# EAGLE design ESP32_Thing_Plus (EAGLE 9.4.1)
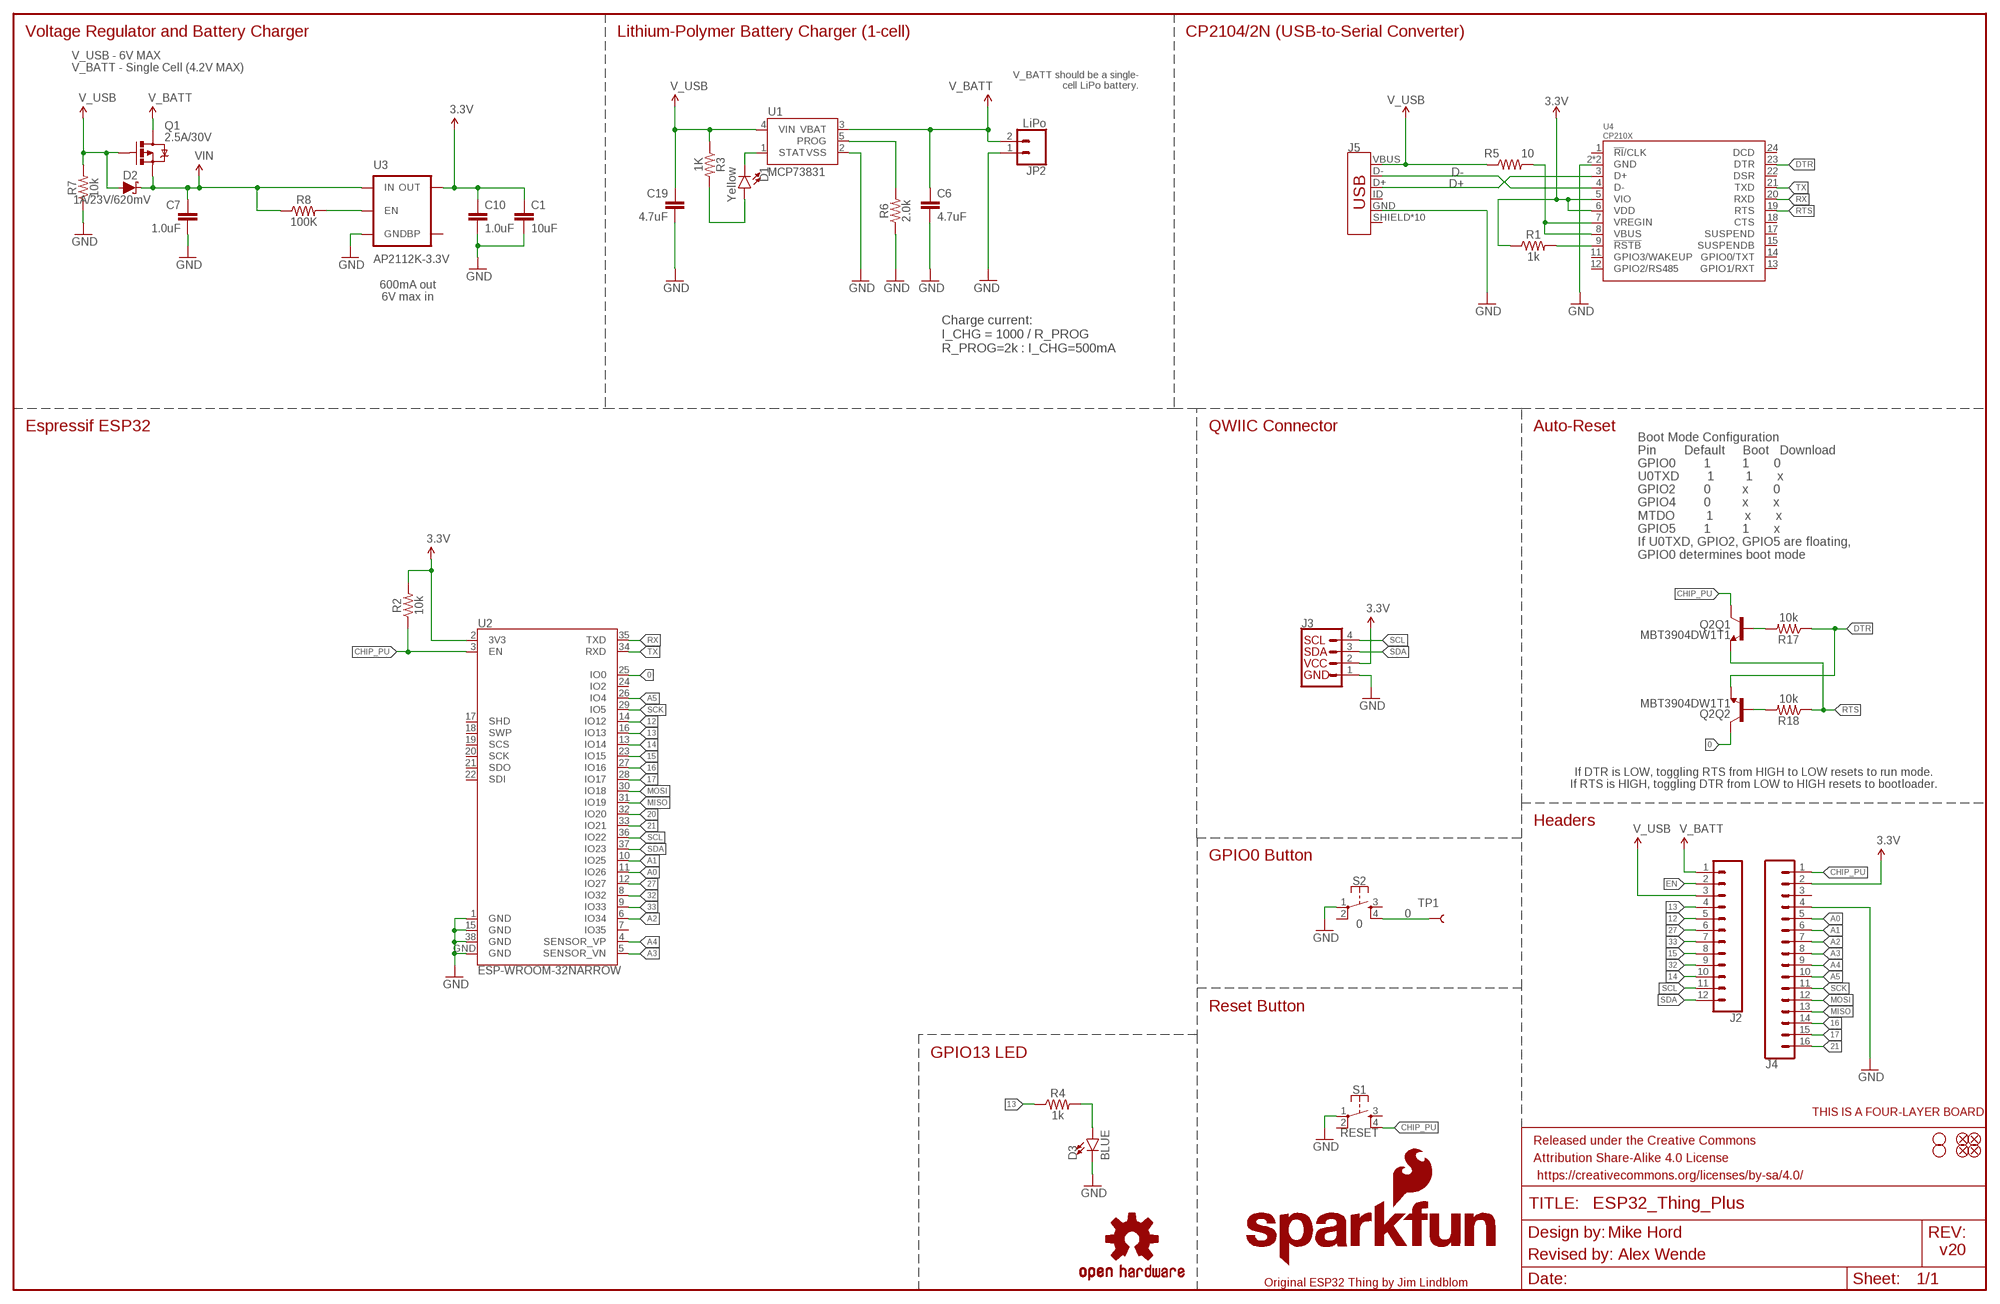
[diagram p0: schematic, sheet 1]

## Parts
C1  10uF  10UF-0603-6.3V-20%  [0603]
C6  4.7uF  4.7UF0603  [0603]
C7  1.0uF  1.0UF-0603-16V-10%-X7R  [0603]
C10  1.0uF  1.0UF-0402-16V-10%  [0402]
C19  4.7uF  4.7UF0603  [0603]
D1  Yellow  LED-YELLOW0603  [LED-0603]
D2  1A/23V/620mV  DIODE-SCHOTTKY-BAT20J  [SOD-323]
D3  BLUE  LED-BLUE0603  [LED-0603]
FD1  FIDUCIALUFIDUCIAL  [FIDUCIAL-MICRO]
FD2  FIDUCIALUFIDUCIAL  [FIDUCIAL-MICRO]
FD3  FIDUCIALUFIDUCIAL  [FIDUCIAL-MICRO]
FD4  FIDUCIALUFIDUCIAL  [FIDUCIAL-MICRO]
FRAME1  FRAME-LEDGER  [CREATIVE_COMMONS]
H1  STAND-OFFTIGHT  [STAND-OFF-TIGHT]
H2  STAND-OFFTIGHT  [STAND-OFF-TIGHT]
J2  CONN_12SM_SQ_NO_SILK  [1X12_SM_SQ_NOSILK]
J3  QWIIC_CONNECTORJS-1MM  [1X04_1MM_RA]
J4  CONN_161X16_SM_SQ_NOSILK  [1X16_SM_SQ_NOSILK]
J5  USB_MICRO-B_HALF_PTH_MILL  [USB-MICROB-PTH-MILL]
JP2  LiPo  CONN_02-JST-2MM-SMT  [JST-2-SMD]
LOGO1  SFE_LOGO_FLAME.1_INCH  [SFE_LOGO_FLAME_.1]
LOGO2  OSHW-LOGOMINI  [OSHW-LOGO-MINI]
LOGO3  SFE_LOGO_NAME_FLAME.1_INCH  [SFE_LOGO_NAME_FLAME_.1]
LOGO4  FOUR_LAYER_WARNING  [FOUR_LAYER_WARNING]
Q1  2.5A/30V  MOSFET-PCHANNELDMG2307L  [SOT23-3@1]
Q2  MBT3904DW1T1  TRANS_NPN_DUAL-MBT3904DW1T1  [SC70-6]
R1  1k  1KOHM-0603-1/10W-1%  [0603]
R2  10k  10KOHM-0603-1/10W-1%  [0603]
R3  1K  1KOHM-1/10W-1%(0603)  [0603]
R4  1k  1KOHM-0603-1/10W-1%  [0603]
R5  10  10OHM-0603-1/10W-5%  [0603]
R6  2.0k  2.0KOHM1/10W5%(0603)  [0603]
R7  10k  10KOHM-0603-1/10W-1%  [0603]
R8  100K  100KOHM-0402-1/16W-1%  [0402]
R17  10k  10KOHM-0603-1/10W-1%  [0603]
R18  10k  10KOHM-0603-1/10W-1%  [0603]
S1  RESET  MOMENTARY-SWITCH-SPST-2-SMD-4.6X2.8MM  [TACTILE_SWITCH_SMD_4.6X2.8MM]
S2  0  MOMENTARY-SWITCH-SPST-2-SMD-4.6X2.8MM  [TACTILE_SWITCH_SMD_4.6X2.8MM]
TP1  TEST-POINTTP_15TH_THRU  [TP_15TH]
U1  MCP73831  [SOT23-5]
U2  ESP-WROOM-32NARROW  [ESP-WROOM-32-NARROW]
U3  AP2112K-3.3V  V_REG_LDOSMD  [SOT23-5]
U4  CP210X  CP2102N  [QFN24]

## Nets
0: Q2.6(Q2:C) S2.4 TP1.P$1 U2.25(IO0)
3.3V: C1.1 C10.1 J3.2 J4.2 R1.1 R2.2 U2.2(3V3) U3.5(OUT) U4.5(VIO) U4.6(VDD)
12: J2.5 U2.14(IO12)
13: J2.4 R4.1 U2.16(IO13)
14: J2.10 U2.13(IO14)
15: J2.8 U2.23(IO15)
16: J4.14 U2.27(IO16)
17: J4.15 U2.28(IO17)
20: U2.32(IO20)
21: J4.16 U2.33(IO21)
27: J2.6 U2.12(IO27)
32: J2.9 U2.8(IO32)
33: J2.7 U2.9(IO33)
A0: J4.5 U2.11(IO26)
A1: J4.6 U2.10(IO25)
A2: J4.7 U2.6(IO34)
A3: J4.8 U2.5(SENSOR_VN)
A4: J4.9 U2.4(SENSOR_VP)
A5: J4.10 U2.26(IO4)
CHG: D1.C U1.1(STAT)
CHIP_PU: J4.1 Q2.3(Q1:C) R2.1 S1.4 U2.3(EN)
D+: J5.D+ U4.3(D+)
D-: J5.D- U4.4(D-)
DTR: Q2.1(Q2:E) R17.1 U4.23(DTR)
EN: J2.2 R8.2 U3.3(EN)
GND: C1.2 C6.2 C7.2 C10.2 C19.2 D3.C J3.1 J4.4 J5.GND JP2.1 R6.1 R7.1 S1.1 S2.1 U1.2(VSS) U2.1(GND) U2.15(GND) U2.38(GND) U2.GND U3.2(GND) U4.2(GND) U4.PAD(GND)
MISO: J4.13 U2.31(IO19)
MOSI: J4.12 U2.30(IO18)
N$1: R1.2 U4.9(!RSTB)
N$2: D3.A R4.2
N$3: R5.2 U4.7(VREGIN) U4.8(VBUS)
N$10: Q2.5(Q1:B) R17.2
N$12: Q2.2(Q2:B) R18.2
N$14: R6.2 U1.5(PROG)
N$17: D1.A R3.2
RTS: Q2.4(Q1:E) R18.1 U4.19(RTS)
RX: U2.35(TXD) U4.20(RXD)
SCK: J4.11 U2.29(IO5)
SCL: J2.11 J3.4 U2.36(IO22)
SDA: J2.12 J3.3 U2.37(IO23)
TX: U2.34(RXD) U4.21(TXD)
V_BATT: C6.1 J2.1 JP2.2 Q1.3(D) U1.3(VBAT)
V_USB: C19.1 D2.A J2.3 J5.VBUS Q1.1(G) R3.1 R5.1 R7.2 U1.4(VIN)
VIN: C7.1 D2.C Q1.2(S) R8.1 U3.1(IN)
Unconnected: J4.3 J5.ID J5.SHIELD J5.SHIELD2(SHIELD) J5.SHIELD3(SHIELD) J5.SHIELD4(SHIELD) J5.SHIELD5(SHIELD) J5.SHIELD6(SHIELD) J5.SHIELD7(SHIELD) J5.SHIELD8(SHIELD) J5.SHIELD9(SHIELD) J5.SHIELD10(SHIELD) S1.2 S1.3 S2.2 S2.3 U2.7(IO35) U2.17(SHD) U2.18(SWP) U2.19(SCS) U2.20(SCK) U2.21(SDO) U2.22(SDI) U2.24(IO2) U3.4(BP) U4.1(!RI!/CLK) U4.11(GPIO3/WAKEUP) U4.12(GPIO2/RS485) U4.13(GPIO1/RXT) U4.14(GPIO0/TXT) U4.15(SUSPENDB) U4.17(SUSPEND) U4.18(CTS) U4.22(DSR) U4.24(DCD)

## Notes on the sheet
- Voltage Regulator and Battery Charger | Lithium-Polymer Battery Charger (1-cell) | CP2104/2N (USB-to-Serial Converter)
- V_USB - 6V MAX
  V_BATT - Single Cell (4.2V MAX)
- V_BATT should be a single-
  cell LiPo battery.
- 600mA out
  6V max in
- Charge current:
  I_CHG = 1000 / R_PROG
  R_PROG=2k : I_CHG=500mA
- Espressif ESP32 | QWIIC Connector | Auto-Reset
- Boot Mode Configuration
  Pin        Default     Boot   Download
  GPIO0        1         1       0
  U0TXD        1         1       x
  GPIO2        0         x       0
  GPIO4        0         x       x
  MTDO         1         x       x
  GPIO5        1         1       x
  If U0TXD, GPIO2, GPIO5 are floating, 
  GPIO0 determines boot mode
- If DTR is LOW, toggling RTS from HIGH to LOW resets to run mode.
  If RTS is HIGH, toggling DTR from LOW to HIGH resets to bootloader.
- Headers
- GPIO0 Button
- Reset Button
- GPIO13 LED
- Mike Hord
- v20
- Revised by: Alex Wende
- Original ESP32 Thing by Jim Lindblom

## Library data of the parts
C1 = SparkFun-Capacitors:10UF: 10.0µF ceramic capacitors; PROD_ID: CAP-11015
C6 C19 = SparkFun-Capacitors:4.7UF: 4.7µF ceramic capacitors; PROD_ID: CAP-08280
C7 = SparkFun-Capacitors:1.0UF: 1µF ceramic capacitors; PROD_ID: CAP-13930
C10 = SparkFun-Capacitors:1.0UF: 1µF ceramic capacitors; PROD_ID: CAP-12417
D1 = SparkFun-LED:LED-YELLOW: Yellow SMD LED; PROD_ID: DIO-09003
D2 = SparkFun-DiscreteSemi:DIODE-SCHOTTKY: Schottky diode; PROD_ID: DIO-11623
D3 = SparkFun-LED:LED-BLUE: Blue SMD LED; PROD_ID: DIO-08575
FD1-FD4 = SparkFun-Aesthetics:FIDUCIAL: Fiducial Alignment Points
FRAME1 = SparkFun-Aesthetics:FRAME-LEDGER: Schematic Frame - Ledger
H1 H2 = SparkFun-Hardware:STAND-OFF: Stand Off
J2 = SparkFun-Connectors:CONN_12: Multi connection point. Often used as Generic Header-pin footprint for 0.1 inch spaced/style header connections On any of the 0.1 inch spaced packages, you can populate with these: Break Away Headers - Straight (PRT-00116) Break Away Male Headers - Right Angle (PRT-00553) Female Headers (PRT-00115)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
J3 = SparkFun-Connectors:QWIIC_CONNECTOR: SparkFun I2C Standard Qwiic Connector An SMD 1mm pitch JST connector makes it easy and quick (get it? Qwiic?) to connect I2C devices to each other. The Qwiic system enables fast and solderless connection between popular platforms and various sensors and actuators. We carry 200mm, 100mm, 50mm, and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; PROD_ID: CONN-13694
J4 = SparkFun-Connectors:CONN_16: Multi connection point. Often used as Generic Header-pin footprint for 0.1 inch spaced/style header connections On any of the 0.1 inch spaced packages, you can populate with these: Break Away Headers - Straight (PRT-00116) Break Away Male Headers - Right Angle (PRT-00553) Female Headers (PRT-00115)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
J5 = SparkFun-Connectors:USB_MICRO-B: USB Type Micro-B Connector Male/female and PTH/SMT variants SparkFun Products: SparkFun microB USB Breakout SparkFun USB microB Plug Breakout SparkFun ESP8266 Thing; PROD_ID: CONN-13711
JP2 = SparkFun-Connectors:CONN_02: Multi connection point. Often used as Generic Header-pin footprint for 0.1 inch spaced/style header connections; PROD_ID: CONN-11443
LOGO1 = SparkFun-Aesthetics:SFE_LOGO_FLAME: SparkFun Flame Logo
LOGO2 = SparkFun-Aesthetics:OSHW-LOGO: Open-Source Hardware (OSHW) Logo
LOGO3 = SparkFun-Aesthetics:SFE_LOGO_NAME_FLAME: SparkFun Font Logo w/ Flame
LOGO4 = SparkFun-Aesthetics:FOUR_LAYER_WARNING: Four-Layer Board Warning - tDoc Layer
Q1 = SparkFun-DiscreteSemi:MOSFET-PCHANNEL: Generic PMOSFET IRLML2244 - TRANS-11153 (SOT-23 -20V -4.3A) (1.Gate 2.Source 3.Drain) FQP27P06 - COM-10349 (TO-220 -60V -27A) (1.Gate 2.Source 3.Drain); PROD_ID: TRANS-11308
Q2 = SparkFun-DiscreteSemi:TRANS_NPN_DUAL: Dual NPN Transistors in Single Package The MBT3904W1 puts two general purpose 3904 NPN transistors in a single package. Datasheet SparkFun Products: SparkFun ESP32 Thing; PROD_ID: TRANS-13337
R1 R4 = SparkFun-Resistors:1KOHM: 1kΩ resistor; PROD_ID: RES-07856
R2 R7 R17 R18 = SparkFun-Resistors:10KOHM: 10kΩ resistor; PROD_ID: RES-00824
R3 = SparkFun-Resistors:1KOHM-1/10W-1%(0603): RES-07856; PROD_ID: RES-07856
R5 = SparkFun-Resistors:10OHM: 10Ω resistor; PROD_ID: RES-09834
R6 = SparkFun-Resistors:2.0KOHM1/10W5%(0603): RES-08296; PROD_ID: RES-08296
R8 = SparkFun-Resistors:100KOHM: 100kΩ resistor; PROD_ID: RES-13495
S1 S2 = SparkFun-Switches:MOMENTARY-SWITCH-SPST-2: Momentary Switch (Pushbutton) - SPST - Two Circuits Normally-open (NO) SPST momentary switches (buttons, pushbuttons). Schematic symbol includes two switch circuits. Variants SMD-4.6MMX2.8MM - 4.60mm x 2.80mm Tactile Momentary Button Switch - Used on SparkFun SAMD21 Mini Breakout SMD-5.2MM - Mini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; PROD_ID: SWCH-13065
TP1 = SparkFun-Connectors:TEST-POINT: SparkFun Test Points
U1 = SparkFun-PowerIC:MCP73831: Miniature single cell, fully integrated Li-Ion, Li-polymer charge management controller http://ww1.microchip.com/downloads/en/DeviceDoc/20001984g.pdf IC-09995; PROD_ID: IC-09995
U2 = SparkFun-RF:ESP-WROOM-32; PROD_ID: IC-13849
U3 = SparkFun-PowerIC:V_REG_LDO: Voltage Regulator LDO Standard 150mA LDO voltage regulator in SOT-23 layout. Micrel part MIC5205. BP (by-pass) pin is used to lower output noise with 470pF cap.; PROD_ID: VREG-12457
U4 = SparkFun-IC-Comms:CP2102N; PROD_ID: IC-14020

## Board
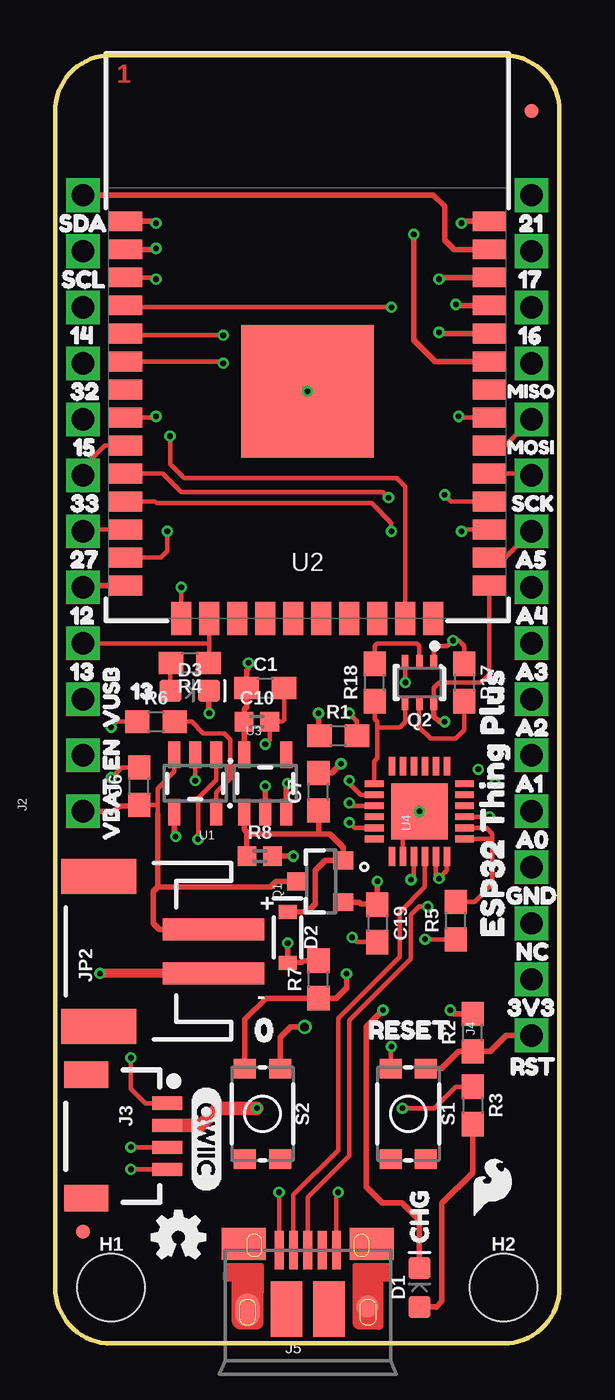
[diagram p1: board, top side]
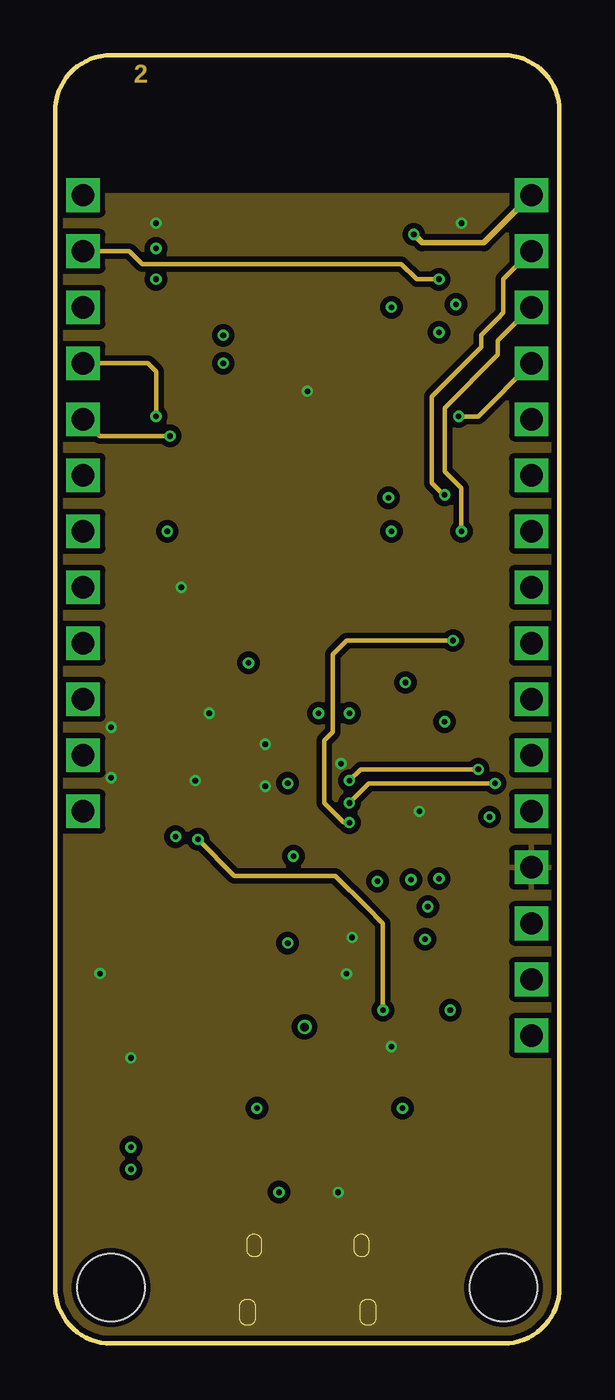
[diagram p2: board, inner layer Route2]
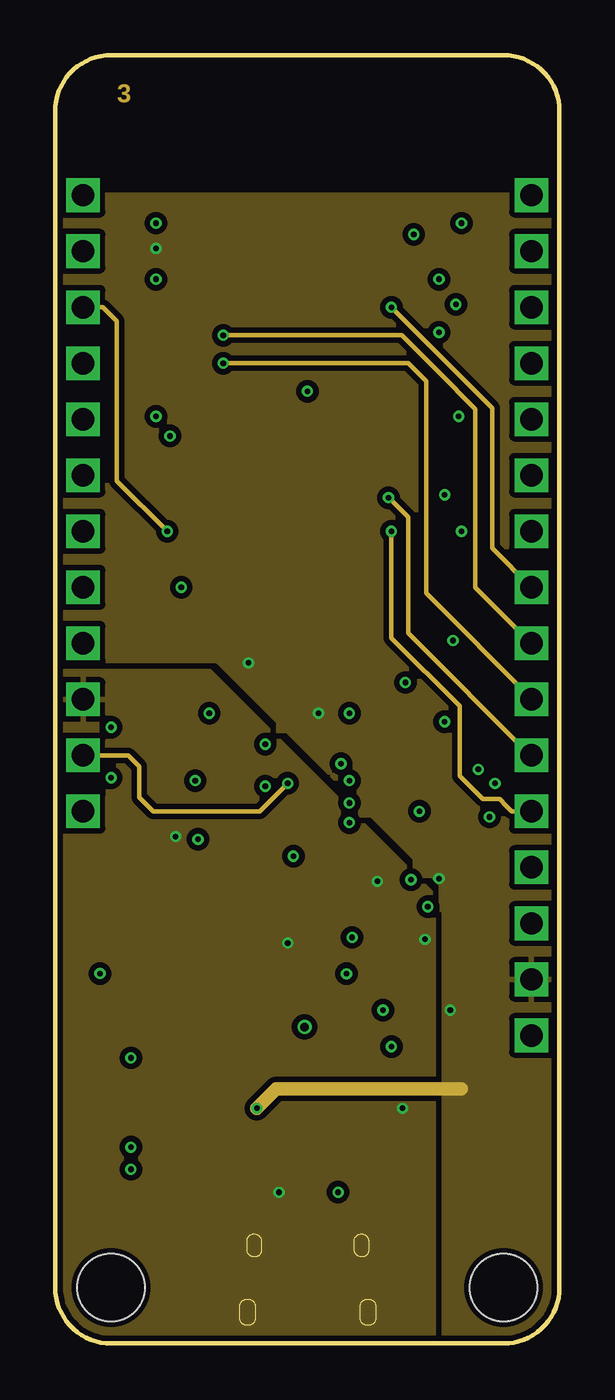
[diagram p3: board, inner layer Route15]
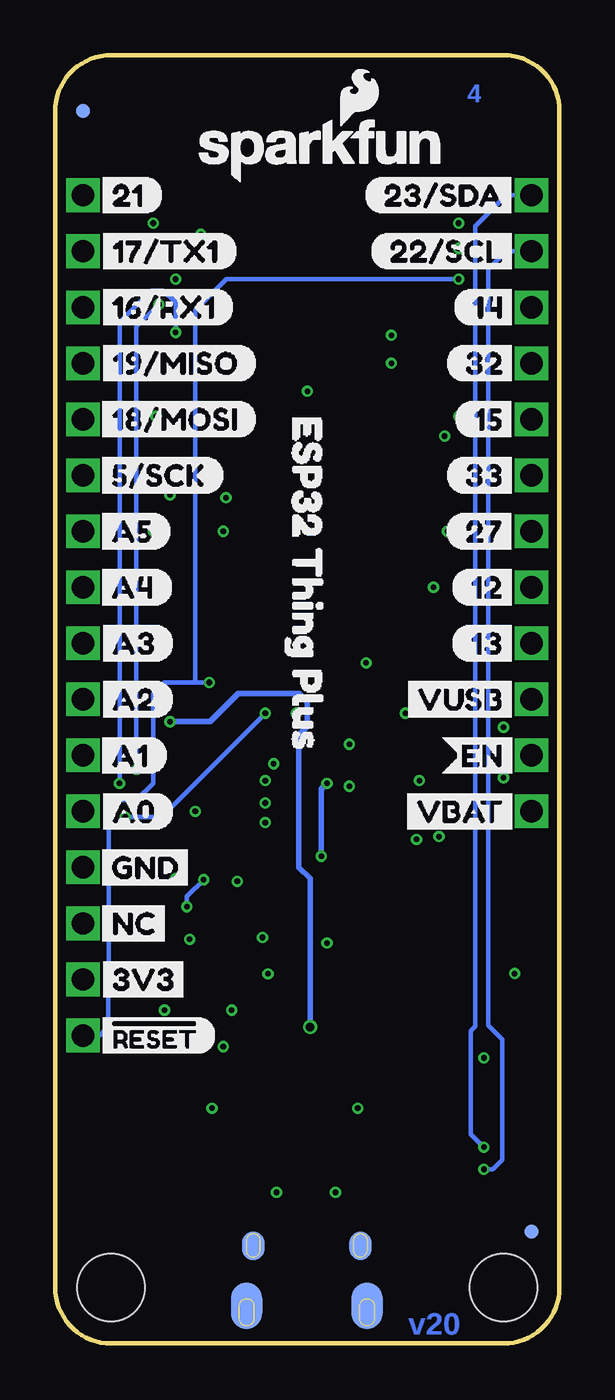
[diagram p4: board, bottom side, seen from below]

Size 22.86 x 58.42 mm. Coordinates in mm from the lower left corner, seen from the top.
Outline: 22.86,2.54 22.86,55.88 arc90 20.32,58.42 2.54,58.42 arc90 0,55.88 0,2.54 arc90 2.54,0 20.32,0 arc90 22.86,2.54
Copper layers (1*2*15*16): Top 0.035559375mm / dielectric 0.47751875mm / Route2 0.035559375mm / dielectric 0.47751875mm / Route15 0.035559375mm / dielectric 0.47751875mm / Bottom 0.035559375mm
Design rules "SparkFun-4-layer-FAB-LIMIT": minimum track width 4mil, minimum drill 6mil, track to track 5mil, track to pad 5mil, pad to pad 5mil, via to via 5mil, smd to smd 5mil, copper to edge 4mil, drill to drill 4mil, minimum pad ring 5mil, minimum via ring 5mil, stop-mask expansion 4mil, vias tented up to drill 25mil, thermal gap 10mil

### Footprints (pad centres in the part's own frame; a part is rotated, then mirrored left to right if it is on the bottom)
0603 = smd 1.1 x 1: 1 -0.85,0; 2 0.85,0
0402 = smd 0.85 x 0.9: 1 -0.58,0; 2 0.58,0
LED-0603 = smd 1 x 1: A -0.877,0; C 0.877,0
SOD-323 = smd 0.63 x 0.83: A 1.15,0; C -1.15,0
FIDUCIAL-MICRO = smd 0.635 x 0.635: 1 0,0
STAND-OFF-TIGHT = hole 3.048: 0,0
1X12_SM_SQ_NOSILK = drill 1.016 pad 1.27 square: 1 0,0; 2 2.54,0; 3 5.08,0; 4 7.62,0; 5 10.16,0; 6 12.7,0; 7 15.24,0; 8 17.78,0; 9 20.32,0; 10 22.86,0; 11 25.4,0; 12 27.94,0
1X04_1MM_RA = smd 0.6 x 1.35: 1 -1.5,0; 2 -0.5,0; 3 0.5,0; 4 1.5,0 | smd 1.2 x 2: NC1 2.8,-3.675; NC2 -2.8,-3.675
1X16_SM_SQ_NOSILK = drill 1.016 pad 1.27 square: 1 0,0; 2 2.54,0; 3 5.08,0; 4 7.62,0; 5 10.16,0; 6 12.7,0; 7 15.24,0; 8 17.78,0; 9 20.32,0; 10 22.86,0; 11 25.4,0; 12 27.94,0; 13 30.48,0; 14 33.02,0; 15 35.56,0; 16 38.1,0
USB-MICROB-PTH-MILL = smd 0.4 x 1.75: D+ 0,0; D- -0.65,0; GND 1.3,0; ID 0.65,0; VBUS -1.3,0 | smd 2 x 1.46: SHIELD -2.9,0.275; SHIELD2 2.9,0.275 | smd 1.425 x 2.5: SHIELD3 -0.963,-2.675; SHIELD4 0.963,-2.675 | smd 1.4 x 2.1 bottom: SHIELD5 -2.731,-2.531; SHIELD7 2.729,-2.531 | smd 1 x 1: SHIELD6 2.7,-2.575 | smd 1.1 x 1.5: SHIELD8 -2.731,-2.731 | smd 1 x 1.3 bottom: SHIELD9 -2.43,0.195; SHIELD10 2.43,0.195
JST-2-SMD = smd 1 x 4.6: 1 -1,-3.7; 2 1,-3.7 | smd 1.6 x 3.4: NC1 -3.4,1.5; NC2 3.4,1.5
SOT23-3@1 = smd 0.8 x 0.9: 1 -0.95,-1; 2 0.95,-1; 3 0,1.1
SC70-6 = smd 0.3 x 0.66: 1 -0.65,-0.92; 2 0,-0.92; 3 0.65,-0.92; 4 0.65,0.92; 5 0,0.92; 6 -0.65,0.92
TACTILE_SWITCH_SMD_4.6X2.8MM = smd 0.9 x 1: 1 -2.05,-0.8; 2 2.05,-0.8; 3 2.05,0.8; 4 -2.05,0.8
TP_15TH = drill 0.381 pad 0.61: P$1 0,0
SOT23-5 = smd 0.55 x 1.2: 1 -0.95,-1.3; 2 0,-1.3; 3 0.95,-1.3; 4 0.95,1.3; 5 -0.95,1.3
ESP-WROOM-32-NARROW = smd 0.9 x 1.5: 1 6.43,8.238; 2 5.16,8.238; 3 3.89,8.238; 4 2.62,8.238; 5 1.35,8.238; 6 0.08,8.238; 7 -1.19,8.238; 8 -2.46,8.238; 9 -3.73,8.238; 10 -5,8.238; 11 -6.27,8.238; 12 -7.54,8.238; 13 -8.81,8.238; 14 -10.08,8.238; 25 -10.08,-8.238; 26 -8.81,-8.238; 27 -7.54,-8.238; 28 -6.27,-8.238; 29 -5,-8.238; 30 -3.73,-8.238; 31 -2.46,-8.238; 32 -1.19,-8.238; 33 0.08,-8.238; 34 1.35,-8.238; 35 2.62,-8.238; 36 3.89,-8.238; 37 5.16,-8.238; 38 6.43,-8.238 | smd 1.5 x 0.9: 15 -11.57,5.715; 16 -11.57,4.445; 17 -11.57,3.175; 18 -11.57,1.905; 19 -11.57,0.635; 20 -11.57,-0.635; 21 -11.57,-1.905; 22 -11.57,-3.175; 23 -11.57,-4.445; 24 -11.57,-5.715 | smd 6 x 6: GND -1.27,0
QFN24 = smd 0.85 x 0.3: 1 -2.05,1.25; 2 -2.05,0.75; 3 -2.05,0.25; 4 -2.05,-0.25; 5 -2.05,-0.75; 6 -2.05,-1.25; 13 2.05,-1.25; 14 2.05,-0.75; 15 2.05,-0.25; 16 2.05,0.25; 17 2.05,0.75; 18 2.05,1.25 | smd 0.3 x 0.85: 7 -1.25,-2.05; 8 -0.75,-2.05; 9 -0.25,-2.05; 10 0.25,-2.05; 11 0.75,-2.05; 12 1.25,-2.05; 19 1.25,2.05; 20 0.75,2.05; 21 0.25,2.05; 22 -0.25,2.05; 23 -0.75,2.05; 24 -1.25,2.05 | smd 2.55 x 2.55: PAD 0,0

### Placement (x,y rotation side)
C1  9.53,29.72 0 top
C6  3.81,25.27 90 top
C7  11.94,25.02 90 top
C10  9.14,28.19 0 top
C19  14.61,19.05 270 top
D1  16.51,2.54 90 top
D2  10.54,18.41 270 top
D3  6.1,29.59 0 top
FD1  21.59,55.88 0 top
FD2  21.59,55.88 0 bottom
FD3  1.27,5.08 0 top
FD4  1.27,5.08 0 bottom
FRAME1  not placed on the board
H1  2.54,2.54 0 top
H2  20.32,2.54 0 top
J2  1.27,24.13 90 top
J3  5.08,9.4 270 top
J4  21.59,13.97 90 top
J5  11.45,4.24 0 top
JP2  3.48,17.78 90 top
LOGO1  18.67,5.46 0 top
LOGO2  5.59,4.83 0 top
LOGO3  16.76,52.58 0 bottom
LOGO4  not placed on the board
Q1  12.06,20.95 90 top
Q2  16.51,29.97 180 top
R1  12.83,27.56 0 top
R2  18.92,14.1 90 top
R3  18.92,10.79 270 top
R4  6.1,30.86 180 top
R5  18.16,19.18 90 top
R6  4.57,28.19 0 top
R7  11.94,16.51 90 top
R8  9.27,22.1 0 top
R17  18.54,29.97 270 top
R18  14.48,29.97 90 top
S1  16,10.41 270 top
S2  9.4,10.41 270 top
TP1  11.3,14.35 0 top
U1  6.35,25.4 180 top
U2  11.43,44.45 90 top
U3  9.53,25.4 0 top
U4  16.51,24.13 90 top
U$1  [#RESET0]  21.34,13.97 0 bottom
U$2  [3V31]  21.21,16.51 0 bottom
U$3  [1323]  4.93,31.75 0 bottom
U$4  [1417]  4.88,46.99 0 bottom
U$5  [1519]  4.83,41.91 0 bottom
U$6  [16#RX11]  21.21,46.99 0 bottom
U$7  [17#TX10]  21.21,49.53 0 bottom
U$8  [121]  4.93,34.29 0 bottom
U$9  [210]  21.18,52.07 0 bottom
U$10  [2721]  5.18,36.83 0 bottom
U$11  [3218]  5.21,44.45 0 bottom
U$12  [3320]  5.21,39.37 0 bottom
U$13  [A03]  21.21,24.13 0 bottom
U$14  [A14]  21.21,26.67 0 bottom
U$15  [A25]  21.21,29.21 0 bottom
U$16  [A36]  21.21,31.75 0 bottom
U$17  [A47]  21.21,34.29 0 bottom
U$18  [A58]  21.21,36.83 0 bottom
U$19  [EN26]  5.38,26.67 0 bottom
U$20  [GND2]  21.21,21.59 0 bottom
U$21  [22#SCL1]  8.64,49.53 0 bottom
U$22  [23#SDA0]  8.86,52.07 0 bottom
U$23  [QWIIC27]  6.86,11.68 270 top
U$27  [VBAT25]  7.39,24.13 0 bottom
U$28  [VUSB24]  7.37,29.21 0 bottom
U$29  [SDA1]  -0.51,50.8 0 top
U$30  [SCL0]  -0.38,48.26 0 top
U$31  [142]  0,45.72 0 top
U$32  [323]  0,43.18 0 top
U$33  [154]  0,40.64 0 top
U$34  [335]  0,38.1 0 top
U$35  [276]  0,35.56 0 top
U$36  [127]  0,33.02 0 top
U$37  [138]  0,30.48 0 top
U$38  [219]  20.19,50.8 0 top
U$39  [1710]  20.32,48.26 0 top
U$40  [1611]  20.32,45.72 0 top
U$41  [A515]  20.19,35.56 0 top
U$42  [A416]  20.07,33.02 0 top
U$43  [A317]  20.07,30.48 0 top
U$44  [A218]  20.07,27.94 0 top
U$45  [A119]  20.19,25.4 0 top
U$46  [A020]  20.19,22.86 0 top
U$47  [SCK20]  20.07,38.1 0 top
U$48  [GND21]  19.76,20.32 0 top
U$49  [NC22]  20.19,17.78 0 top
U$50  [VUSB8]  2.54,27.3 90 top
U$51  [EN9]  2.54,25.4 90 top
U$52  [VBAT10]  2.54,22.23 90 top
U$53  [137]  2.79,29.59 0 top
U$54  [MISO0]  19.94,43.18 0 top
U$55  [MOSI1]  19.94,40.64 0 top
U$56  [CHG1]  16.51,3.81 90 top
U$57  [RESET0]  13.46,14.22 0 top
U$58  [ESP32_THING_PLUS0]  19.81,17.53 90 top
U$59  [ORDERING_INSTRUCTIONS]  not placed on the board
U$60  [3V323]  19.81,15.24 0 top
U$61  [RST24]  19.94,12.57 0 top
U$62  [00]  8.13,14.22 0 top
U$63  [5#SCK2]  21.21,39.37 0 bottom
U$64  [NC0]  21.21,19.05 0 bottom
U$65  [ESP32_THING_PLUS0]  11.43,43.18 270 bottom
U$66  [18#MOSI1]  21.21,41.91 0 bottom
U$67  [19#MISO0]  21.21,44.45 0 bottom

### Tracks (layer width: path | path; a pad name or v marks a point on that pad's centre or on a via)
0  (via drill 0.25)
  Top 0.203: U2.25 19.67,30.34 19.3,29.97 17.4,29.97 17.16,29.73 Q2.6
  Top 0.254: S2.4 10.2,13.88 10.67,14.35 TP1.P$1 | v17.65,28.19 17.4,28.19 17.16,28.43 Q2.6
  Bottom 0.254: v17.65,28.19 15.83,28.19 14.56,29.46 11.81,29.46 11.43,29.08 11.43,27.98 11.81,27.6 11.81,21.59 11.3,21.08 TP1.P$1
3.3V  (via drill 0.25)
  Top 0.203: U4.5 17.26,21.22 v17.4,21.08 17.76,21.44 U4.6
  Top 0.254: U2.2 4.53,49.61 v4.57,49.66 | U3.5 8.57,28.18 C10.1 8.56,28.76 8.68,28.87 C1.1 8.68,30.52 8.76,30.61 v8.76,30.86 | R1.1 11.94,27.6 v11.94,28.57 | R2.2 18.07,14.95 v17.91,15.11
  Top 0.61: J3.2 6.6,9.9 7.37,10.67 v9.14,10.67
  Route15 0.61: v9.14,10.67 10.03,11.56 18.41,11.56
  pour Route15 (isolate 0.254, rank 2): 0,52.07 22.86,52.07 22.86,0 0,0
12
  Top 0.254: U2.14 1.35,34.37 J2.5
13
  Top 0.203: U2.16 6.99,31.75 | 6.99,31.75 6.99,30.9 R4.1 | J2.4 6.99,31.75
14  (via drill 0.25)
  Top 0.203: U2.13 4.78,35.64 5.08,35.94 v5.08,36.83
  Route15 0.203: v5.08,36.83 2.79,39.12 2.79,46.35 2.16,46.99 J2.10
15  (via drill 0.25)
  Top 0.203: U2.23 15.88,38.86 15.49,39.24 5.84,39.24 5.21,39.88 v5.21,41.15
  Route2 0.203: v5.21,41.15 2.03,41.15 J2.8
16  (via drill 0.25)
  Top 0.203: U2.27 18.5,36.91 v18.41,36.83
  Route2 0.203: v18.41,36.83 18.41,38.78 17.65,39.54 17.65,42.42 20.07,44.83 20.07,45.47 J4.14
17  (via drill 0.25)
  Top 0.203: U2.28 17.95,38.18 v17.65,38.48
  Route2 0.203: J4.15 20.32,48.26 20.32,46.74 20.07,46.48 19.3,45.72 19.3,45.17 17.07,42.94 17.07,39.02 17.61,38.48 v17.65,38.48
21  (via drill 0.25)
  Top 0.254: v16.26,50.29 16.26,45.5 17.23,44.53 U2.33
  Route2 0.254: J4.16 20.32,50.8 19.43,49.91 16.64,49.91 v16.26,50.29
27
  Top 0.203: U2.12 1.35,36.91 J2.6
32  (via drill 0.25)
  Top 0.203: U2.8 4.53,41.99 v4.57,42.04
  Route2 0.203: v4.57,42.04 4.57,44.07 4.19,44.45 J2.9
33
  Top 0.203: U2.9 2.24,40.72 1.27,39.75 J2.7
A0  (via drill 0.25)
  Top 0.203: U2.11 4.53,38.18 4.61,38.1 14.35,38.1 15.24,37.21 v15.24,36.83
  Route15 0.203: v15.24,36.83 15.24,32 18.34,28.9 18.34,25.73 19.38,24.69 20.14,24.69 20.45,24.38 20.7,24.13 J4.5
A1  (via drill 0.25)
  Top 0.203: U2.10 4.87,39.45 5.71,38.61 14.86,38.61 v15.11,38.35
  Route15 0.203: J4.6 21.55,26.67 16,32.21 16,37.47 v15.11,38.35
A2  (via drill 0.25)
  Top 0.203: U2.6 7.54,44.53 v7.62,44.45
  Route15 0.203: v7.62,44.45 16,44.45 16.82,43.64 16.82,34.03 21.59,29.25 J4.7
A3  (via drill 0.25)
  Top 0.203: U2.5 3.27,45.72 v7.62,45.72
  Route15 0.203: v7.62,45.72 15.71,45.72 17.36,44.07 19.05,42.38 19.05,37.17 19.05,36.49 19.05,34.29 J4.8
A4  (via drill 0.25)
  Top 0.203: U2.4 3.27,46.99 v15.24,46.99
  Route15 0.203: v15.24,46.99 17.53,44.7 19.81,42.42 19.81,36.07 J4.9
A5
  Top 0.203: U2.26 20.4,35.64 J4.10
CHG  (via drill 0.25)
  Top 0.203: U1.1 7.3,25.55 6.48,24.73 v6.48,22.86
  Top 0.254: v14.86,15.11 14.1,14.35 14.1,7.11 14.82,6.39 15.71,6.39 16.51,5.59 D1.C
  Route2 0.203: v6.48,22.86 8.13,21.21 12.7,21.21 14.1,19.81 14.86,19.05 v14.86,15.11
CHIP_PU  (via drill 0.25)
  Top 0.203: U2.3 4.49,48.34 v4.57,48.26 | v15.88,29.97 15.86,29.99 Q2.3
  Top 0.254: S1.4 16.8,12.48 17.53,12.48 18.29,13.25 R2.1 19.72,13.25 20.45,13.97 J4.1
  Bottom 0.203: v15.88,29.97 16.51,29.97 | 16.51,29.97 17.91,29.97 18.41,29.46 18.41,25.4 19.18,24.64 19.94,24.64 20.42,24.16 20.42,16.03 20.45,16 20.45,14.35 20.83,13.97 J4.1 | v4.57,48.26 15.11,48.26 16.51,46.86 16.51,29.97
D+  (via drill 0.25)
  Top 0.203: v16.89,19.81 16.51,19.81 16.13,19.43 16.13,17.44 13.34,14.65 13.34,8.51 11.45,6.62 J5.D+ | v16.13,21.03 16.26,21.16 U4.3
  Bottom 0.203: v16.89,19.81 16.89,20.27 v16.13,21.03
D-
  Top 0.203: U4.4 16.76,20.7 15.62,19.56 15.62,17.53 12.83,14.73 12.83,8.76 10.8,6.74 J5.D-
DTR  (via drill 0.25)
  Top 0.203: R17.1 18.54,31.62 18.29,31.88 v18.03,31.88 17.78,31.62 17.4,31.62 17.16,31.38 Q2.1 | U4.23 13.58,23.38 v13.34,23.62
  Route2 0.203: v18.03,31.88 13.21,31.88 12.57,31.24 12.57,27.94 12.57,27.73 12.19,27.35 12.19,24.51 13.08,23.62 v13.34,23.62
EN  (via drill 0.25)
  Top 0.254: R8.2 v10.79,22.1 | U3.3 10.47,25.33 v10.54,25.4
  Route15 0.203: J2.2 3.3,26.67 3.81,26.16 3.81,24.77 4.45,24.13 9.27,24.13 v10.54,25.4
  Bottom 0.254: v10.79,22.1 10.79,25.15 v10.54,25.4
GND  (via drill 0.25)
  Top 0.203: U1.2 v6.35,25.53 | C1.2 10.38,28.28 10.29,28.19 C10.2 9.72,27.38 v9.53,27.18 | U2.15 v5.71,34.29 | C19.2 13.68,18.2 v13.46,18.41 | C6.2 3.01,26.12 v2.54,25.65 | R6.1 2.79,28.19 v2.54,27.94 | U4.2 15.76,23.38 U4.PAD | J3.1 4.09,10.9 3.43,11.56 v3.43,12.95 | S1.1 15.2,13.46 v15.24,13.46 | v12.83,6.86 12.75,6.78 J5.GND
  Top 0.254: U2.1 4.49,50.88 v4.57,50.8 | U3.2 v9.53,25.27 | D3.C 6.97,28.59 v6.99,28.57 | C7.2 12.53,25.87 v12.95,26.29 | S2.1 8.6,14.69 9.56,15.66 R7.1 12.74,15.66 13.21,16.13 v13.21,16.76 | U2.38 18.5,50.88 v18.41,50.8
  Top 0.406: JP2.1 v2.03,16.78
  other vias: 11.43,43.18 16.51,24.13
  pour Route2 (isolate 0.254): 0,52.07 22.86,52.07 22.86,0 0,0
MISO  (via drill 0.25)
  Top 0.203: U2.31 18.34,41.99 v18.29,42.04
  Route2 0.203: v18.29,42.04 19.18,42.04 J4.13
MOSI
  Top 0.203: U2.30 20.4,40.72 J4.12
N$1  (via drill 0.25)
  Top 0.203: v19.68,23.88 U4.9 | v13.34,28.57 13.68,28.23 R1.2
  Bottom 0.203: v13.34,28.57 13.97,27.94 18.03,23.88 v19.68,23.88
N$2
  Top 0.203: D3.A 5.22,30.83 R4.2
N$3
  Top 0.203: U4.8 19.18,23.38 19.18,23.37 19.56,23.37 19.81,23.11 19.81,22.88 | R5.2 19.01,20.03 19.81,20.83 19.81,22.73 19.81,22.88 | U4.7 19.81,22.88
N$10
  Top 0.203: Q2.5 16.51,27.94 17.02,27.43 17.53,27.43 18.16,27.43 18.54,27.81 R17.2
N$12
  Top 0.203: Q2.2 16.51,31.62 16.38,31.75 14.61,31.75 14.48,31.62 R18.2
N$14
  Top 0.203: U1.5 7.3,24.99 7.93,25.62 7.93,27.39 7.67,27.66 6.72,27.66 6.18,28.19 R6.2
N$17
  Top 0.254: R3.2 18.92,7.75 17.53,6.35 17.53,1.91 17.27,1.65 17.26,1.66 D1.A
RTS
  Top 0.203: U4.19 14.46,26.4 14.61,26.54 14.61,27.94 | 14.61,27.94 14.61,28.19 14.48,28.32 R18.1 | Q2.4 15.86,28.18 15.62,27.94 14.61,27.94
RX  (via drill 0.25)
  Top 0.203: U4.20 13.86,24.88 13.34,25.4 v13.34,25.53
  Top 0.254: U2.35 18.21,47.07 v18.16,47.12
  Route2 0.203: v19.18,26.04 13.84,26.04 v13.34,25.53
  Bottom 0.203: v19.18,26.04 19.18,46.1 v18.16,47.12
SCK
  Top 0.203: U2.29 21.51,39.45 J4.11
SCL  (via drill 0.25)
  Top 0.203: J3.4 v3.43,7.9
  Top 0.254: U2.36 17.48,48.34 v17.4,48.26
  Route2 0.203: J2.11 3.35,49.53 | v17.4,48.26 16.51,48.26 16.38,48.26 15.7,48.95 3.94,48.95 3.35,49.53 | 3.35,49.53 | 3.35,49.53 | 3.35,49.53
  Bottom 0.203: J2.11 2.41,49.53 3.23,48.72 3.23,14.43 2.59,13.79 2.59,8.33 3.02,7.9 3.13,7.9 v3.43,7.9
SDA  (via drill 0.25)
  Top 0.203: J3.3 v3.43,8.9
  Top 0.254: J2.12 17.14,52.07 17.65,51.56 17.65,50.04 18.08,49.61 U2.37
  Bottom 0.203: J2.12 2.41,52.07 3.81,50.67 3.81,14.38 4.01,14.17 4.01,9.48 v3.43,8.9
TX  (via drill 0.25)
  Top 0.203: U4.21 13.47,24.38 v13.34,24.51
  Top 0.254: v17.4,45.85 17.45,45.8 U2.34
  Route2 0.203: v19.94,25.4 14.22,25.4 v13.34,24.51
  Bottom 0.203: v17.4,45.85 17.4,46.65 17.4,47.2 17.95,47.75 18.5,47.75 19.94,46.31 v19.94,25.4
V_BATT
  Top 0.203: 4.64,24.42 4.64,25.18 5.4,25.93 U1.3 | 4.64,24.42 4.64,24 | C6.1 4.64,24.42
  Top 0.254: Q1.3 10.03,20.95 9.78,20.7 5.08,20.7 4.64,20.7 | J2.1 2.67,24.13 2.92,24.38 3.81,24.38 C6.1 | 4.64,20.7 4.64,24 | JP2.2 4.71,18.78 4.45,19.05 4.45,20.5 4.64,20.7
V_USB  (via drill 0.25)
  Top 0.203: v15.75,10.67 17.18,10.67 18.16,11.64 R3.1 | R5.1 v16.76,18.33 | J5.VBUS v10.15,6.86
  Top 0.254: Q1.1 13.78,20 13.84,19.94 14.57,19.94 C19.1 v14.61,20.95 | U1.4 5.4,23.05 v5.46,22.99 | R7.2 11.26,17.36 11.18,17.27 D2.A v10.54,18.16
  pour Route15 (isolate 0.254): 17.14,0 17.14,20.32 6.99,30.48 0,30.48 0,0
VIN
  Top 0.254: D2.C 11.42,19.57 11.8,19.94 11.8,21.45 12.25,21.91 Q1.2 13.06,22.5 12.45,23.11 11.94,23.11 | 11.94,23.11 8.76,23.11 8.69,23.04 | U3.1 8.57,23.3 8.69,23.19 8.69,23.04 | C7.1 11.94,23.11 | R8.1 8.69,22.86 8.69,23.04

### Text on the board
Top: 1
Route2: 2
Route15: 3
Bottom: 4 | v20
tPlace: + | -
Measures: Units in inches
tDocu: Mike Hord | Revised by: Alex Wende

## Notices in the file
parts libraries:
SparkFun-Aesthetics: Licensing: Creative Commons ShareAlike 4.0 International - https://creativecommons.org/licenses/by-sa/4.0
SparkFun-Aesthetics: Released under the Creative Commons Attribution Share-Alike 4.0 License
SparkFun-Aesthetics: https://creativecommons.org/licenses/by-sa/4.0
